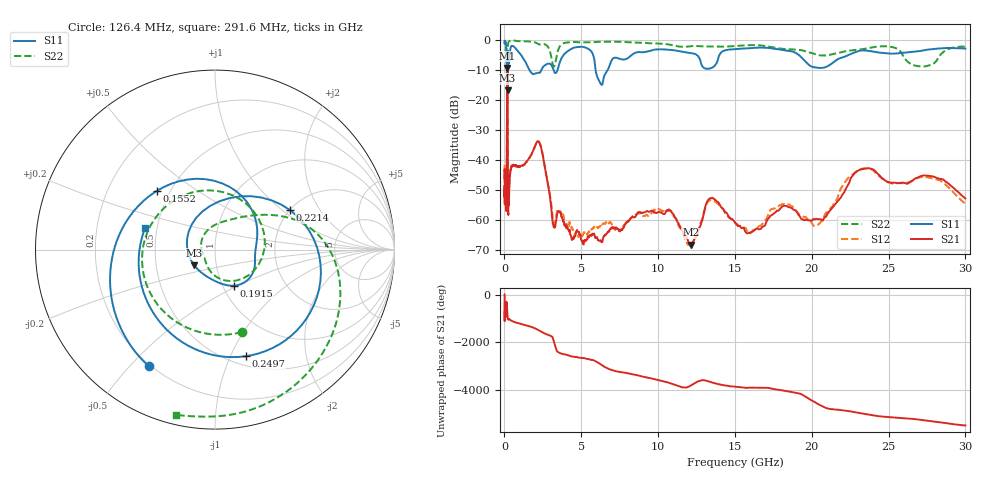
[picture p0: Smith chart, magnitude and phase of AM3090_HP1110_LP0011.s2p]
! Date/Time: Thu, Feb 28, 2019 2:08 PM
! Network Analyzer: Agilent Technologies E8364B Rev: A.07.50.67
! Sweep from 0.010 to 30.000 GHz, 1601 Points, Sweep Type: LOG
! Power Supply: 5.023 V, 0.002 A
# Hz S DB R 50
!freq MagS11 AngS11 MagS21 AngS21 MagS12 AngS12 MagS22 AngS22
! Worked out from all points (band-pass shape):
!   1601 points, 10 MHz to 30 GHz, reference 50 ohm
!   highest |S21| = -9.33 dB at 182.2 MHz (marker M1); lowest = -68.4 dB at 12.13 GHz (marker M2)
!   |S21| within 3 dB of the highest: 170.1 MHz to 197 MHz (26.94 MHz wide, 14.7 % of centre)
!   lowest |S11| = -16.8 dB at 202.3 MHz (marker M3), VSWR 1.34, Z = 39.1 - j7.04 ohm
!   |S11| at or under -10 dB: 1.624 GHz to 2.4 GHz (776.2 MHz wide, 38.6 % of centre); 3.201 GHz to 3.455 GHz (254.2 MHz wide, 7.64 % of centre); 5.93 GHz to 6.722 GHz (791.6 MHz wide, 12.5 % of centre)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
!   |S22| runs from -22.9 to -0.2 dB; largest |S21 - S12| = 0.013
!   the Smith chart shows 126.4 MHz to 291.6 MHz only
!   S11 on the Smith chart (normalised r, x): 126.4 MHz: 0.19, -0.57; 155.2 MHz: 0.42, +0.35; 191.5 MHz: 1.13, -0.48; 221.4 MHz: 2.00, +1.14; 249.7 MHz: 0.60, -1.15; 291.6 MHz: 0.43, +0.12
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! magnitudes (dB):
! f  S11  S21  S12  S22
! 10 MHz  -0.3  -46.0  -41.7  -0.6
! 38.04 MHz  -0.3  -51.5  -51.1  -1.2
! 126.4 MHz  -2.5  -56.9  -54.2  -6.3
! 144.7 MHz  -4.5  -48.6  -47.7  -8.3
! 155.2 MHz  -6.7  -31.3  -31.5  -10.2
! 182.2 MHz  -12.4  -9.3  -9.3  -22.3
! 191.5 MHz  -12.9  -10.3  -10.3  -16.9
! 202.3 MHz  -16.8  -16.4  -16.4  -10.5
! 221.4 MHz  -6.5  -44.8  -46.3  -2.6
! 249.7 MHz  -4.2  -58.3  -53.5  -0.9
! 291.6 MHz  -7.8  -53.0  -53.2  -0.5
! 550.5 MHz  -2.1  -41.7  -41.9  -0.2
! 2.084 GHz  -11.1  -34.3  -34.3  -1.0
! 3.236 GHz  -10.5  -62.6  -61.3  -8.8
! 7.926 GHz  -6.3  -61.1  -61.1  -0.7
! 10.44 GHz  -3.2  -58.1  -57.3  -1.3
! 12.13 GHz  -4.4  -68.4  -68.9  -2.1
! 13.54 GHz  -9.2  -52.7  -53.5  -2.2
! 15.73 GHz  -2.8  -64.4  -63.0  -1.8
! 20.31 GHz  -9.2  -59.7  -61.7  -4.9
! 23.36 GHz  -3.5  -43.1  -42.9  -3.0
! 30 GHz  -2.9  -52.9  -54.7  -2.2
